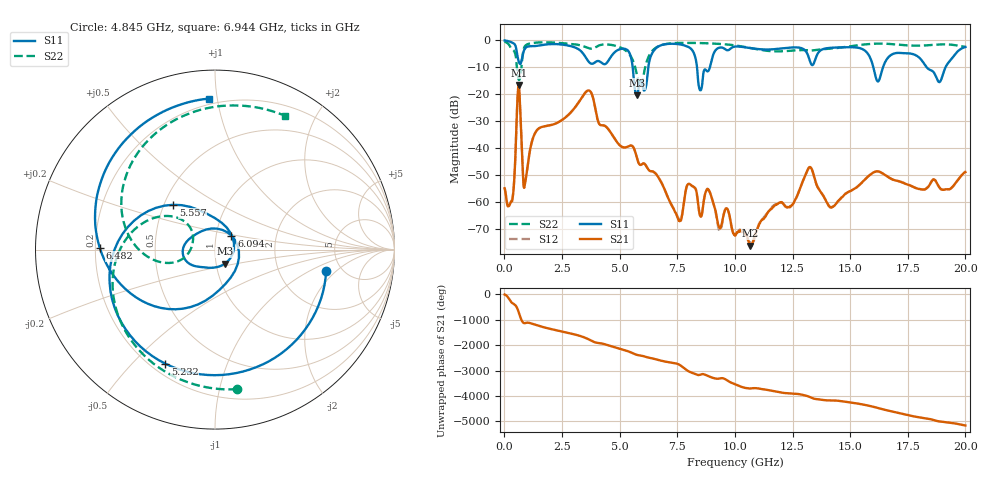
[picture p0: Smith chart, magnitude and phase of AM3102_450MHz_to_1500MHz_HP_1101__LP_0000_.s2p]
!Agilent Technologies,E8364B,MY43040894,A.07.50.67
!Agilent E8364B: A.07.50.67
!Date: Thursday, January 11, 2018 06:37:01
!Correction: S11(Full 2 Port(1,2))
!S21(Full 2 Port(1,2))
!S12(Full 2 Port(1,2))
!S22(Full 2 Port(1,2))
!S2P File: Measurements: S11, S21, S12, S22:
# Hz S  dB  R 50
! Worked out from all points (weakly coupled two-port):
!   1601 points, 10 MHz to 20 GHz, reference 50 ohm
!   highest |S21| = -16.57 dB at 622.2 MHz (marker M1); lowest = -76.2 dB at 10.65 GHz (marker M2)
!   lowest |S11| = -20.3 dB at 5.745 GHz (marker M3), VSWR 1.21, Z = 55 - j8.79 ohm
!   |S11| at or under -10 dB: 5.567 GHz to 6.243 GHz (676.4 MHz wide, 11.5 % of centre); 8.357 GHz to 8.916 GHz (558.7 MHz wide, 6.47 % of centre); 18.32 GHz to 19.14 GHz (819.3 MHz wide, 4.37 % of centre)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
!   |S22| runs from -17.8 to -0.5 dB; largest |S21 - S12| = 0.0018
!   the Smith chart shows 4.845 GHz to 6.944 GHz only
!   S11 on the Smith chart (normalised r, x): 4.845 GHz: 3.78, -1.50; 5.232 GHz: 0.26, -0.63; 5.557 GHz: 0.56, +0.32; 6.094 GHz: 1.18, +0.19; 6.482 GHz: 0.22, +0.01; 6.944 GHz: 0.16, +0.95
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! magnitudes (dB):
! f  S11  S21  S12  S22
! 10 MHz  -0.1  -54.9  -54.8  -0.5
! 334.8 MHz  -0.8  -59.7  -59.0  -3.3
! 622.2 MHz  -7.9  -16.6  -16.6  -14.6
! 897.1 MHz  -3.1  -53.0  -52.9  -2.1
! 1.397 GHz  -2.1  -33.5  -33.5  -0.8
! 3.346 GHz  -4.2  -21.4  -21.4  -2.0
! 4.845 GHz  -4.0  -37.3  -37.3  -2.1
! 5.232 GHz  -3.2  -39.8  -39.8  -3.6
! 5.557 GHz  -9.3  -39.3  -39.3  -7.1
! 5.745 GHz  -20.3  -43.4  -43.5  -12.7
! 6.094 GHz  -18.4  -45.9  -45.9  -10.5
! 6.482 GHz  -3.9  -48.9  -48.8  -3.3
! 6.682 GHz  -2.3  -50.8  -50.7  -2.2
! 6.944 GHz  -1.5  -55.2  -55.1  -1.5
! 8.493 GHz  -18.5  -65.1  -65.3  -1.0
! 10.01 GHz  -2.3  -72.4  -72.1  -1.9
! 10.65 GHz  -2.9  -76.2  -75.0  -2.8
! 13.34 GHz  -9.2  -47.9  -47.9  -3.8
! 14.18 GHz  -2.8  -61.9  -61.9  -3.1
! 16.68 GHz  -6.1  -50.9  -50.8  -1.3
! 18.86 GHz  -15.5  -54.4  -54.5  -1.6
! 20 GHz  -2.5  -48.9  -48.7  -2.4
